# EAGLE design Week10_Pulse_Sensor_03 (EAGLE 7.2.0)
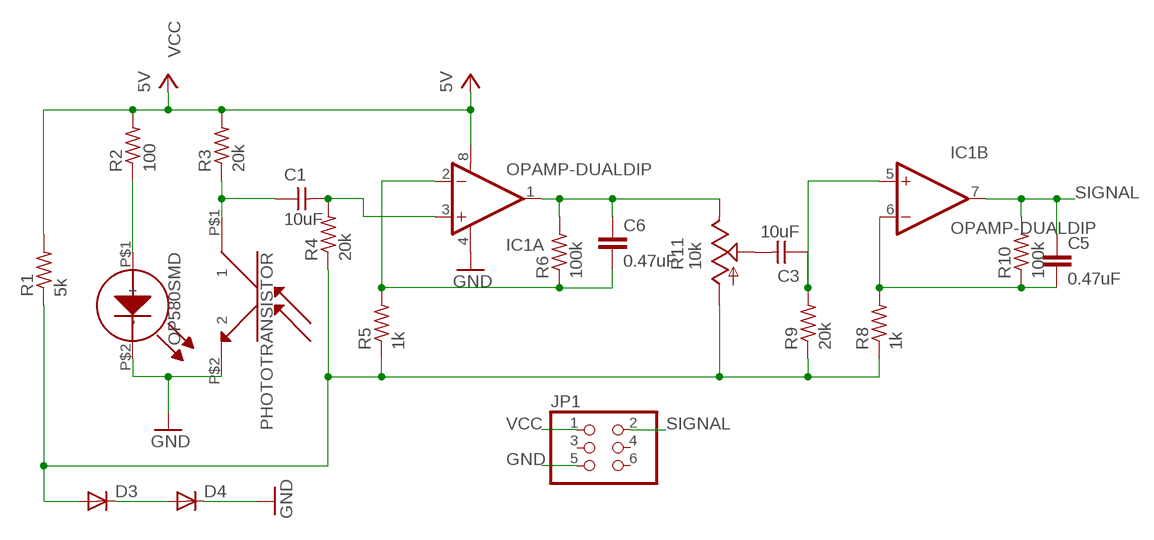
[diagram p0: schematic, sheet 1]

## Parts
C1  10uF  UNPOLARIZED_CAPACITOR1206  [1206]
C3  10uF  UNPOLARIZED_CAPACITOR1206  [1206]
C5  0.47uF  C-EU050-045X075  [C050-045X075]
C6  0.47uF  C-EU050-045X075  [C050-045X075]
D3  DIODESOD123  [SOD123]
D4  DIODESOD123  [SOD123]
IC1  OPAMP-DUALDIP  [DIP08]
JP1  PINHD-2X3-SMD  [2X03SMD]
LED  OP280SMD  [OP280]
PHOTOTRANSISTOR  OP580SMD  [OP580]
R1  5k  RES-US1206FAB  [R1206FAB]
R2  100  RES-US1206FAB  [R1206FAB]
R3  20k  RES-US1206FAB  [R1206FAB]
R4  20k  RES-US1206FAB  [R1206FAB]
R5  1k  RES-US1206FAB  [R1206FAB]
R6  100k  RES-US1206FAB  [R1206FAB]
R8  1k  RES-US1206FAB  [R1206FAB]
R9  20k  RES-US1206FAB  [R1206FAB]
R10  100k  RES-US1206FAB  [R1206FAB]
R11  10k  TRIM_US-S64W  [S64W]

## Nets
GND: D4.CATHODE(C) IC1.4(A:V-) JP1.5 LED.P$2(-) PHOTOTRANSISTOR.P$2
N$1: C1.1 PHOTOTRANSISTOR.P$1 R3.1
N$2: LED.P$1(+) R2.1
N$3: D3.CATHODE(C) D4.ANODE(A)
N$4: C5.2 IC1.6(B:-IN) R8.2 R10.1
N$5: C6.2 IC1.2(A:-IN) R5.2 R6.1
N$6: C1.2 IC1.3(A:+IN) R4.2
N$7: C6.1 IC1.1(A:OUT) R6.2 R11.E
N$8: C3.2 R11.S
N$9: C3.1 IC1.5(B:+IN) R9.2
N$11: D3.ANODE(A) R1.1 R4.1 R5.1 R8.1 R9.1 R11.A
SIGNAL: C5.1 IC1.7(B:OUT) JP1.2 R10.2
VCC: IC1.8(A:V+) JP1.1 R1.2 R2.2 R3.2 ; supply symbol labelled 5V
Unconnected: JP1.3 JP1.4 JP1.6

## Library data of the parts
C1 C3 = 01_ng:UNPOLARIZED_CAPACITOR: unpolarized_capacitor
C5 C6 = rcl:C-EU: CAPACITOR, European symbol
D3 D4 = 01_fab:DIODE: DIODE
IC1 = SparkFun-AnalogIC:OPAMP-DUAL: Generic op-amp footprint
JP1 = 01_FAB_Hello:PINHD-2X3-SMD: PIN HEADER
LED = Optics:OP280
PHOTOTRANSISTOR = Optics:OP580
R1-R6 R8-R10 = 01_fab:RES-US: Resistor (US Symbol)
R11 = pot:TRIM_US-: POTENTIOMETER

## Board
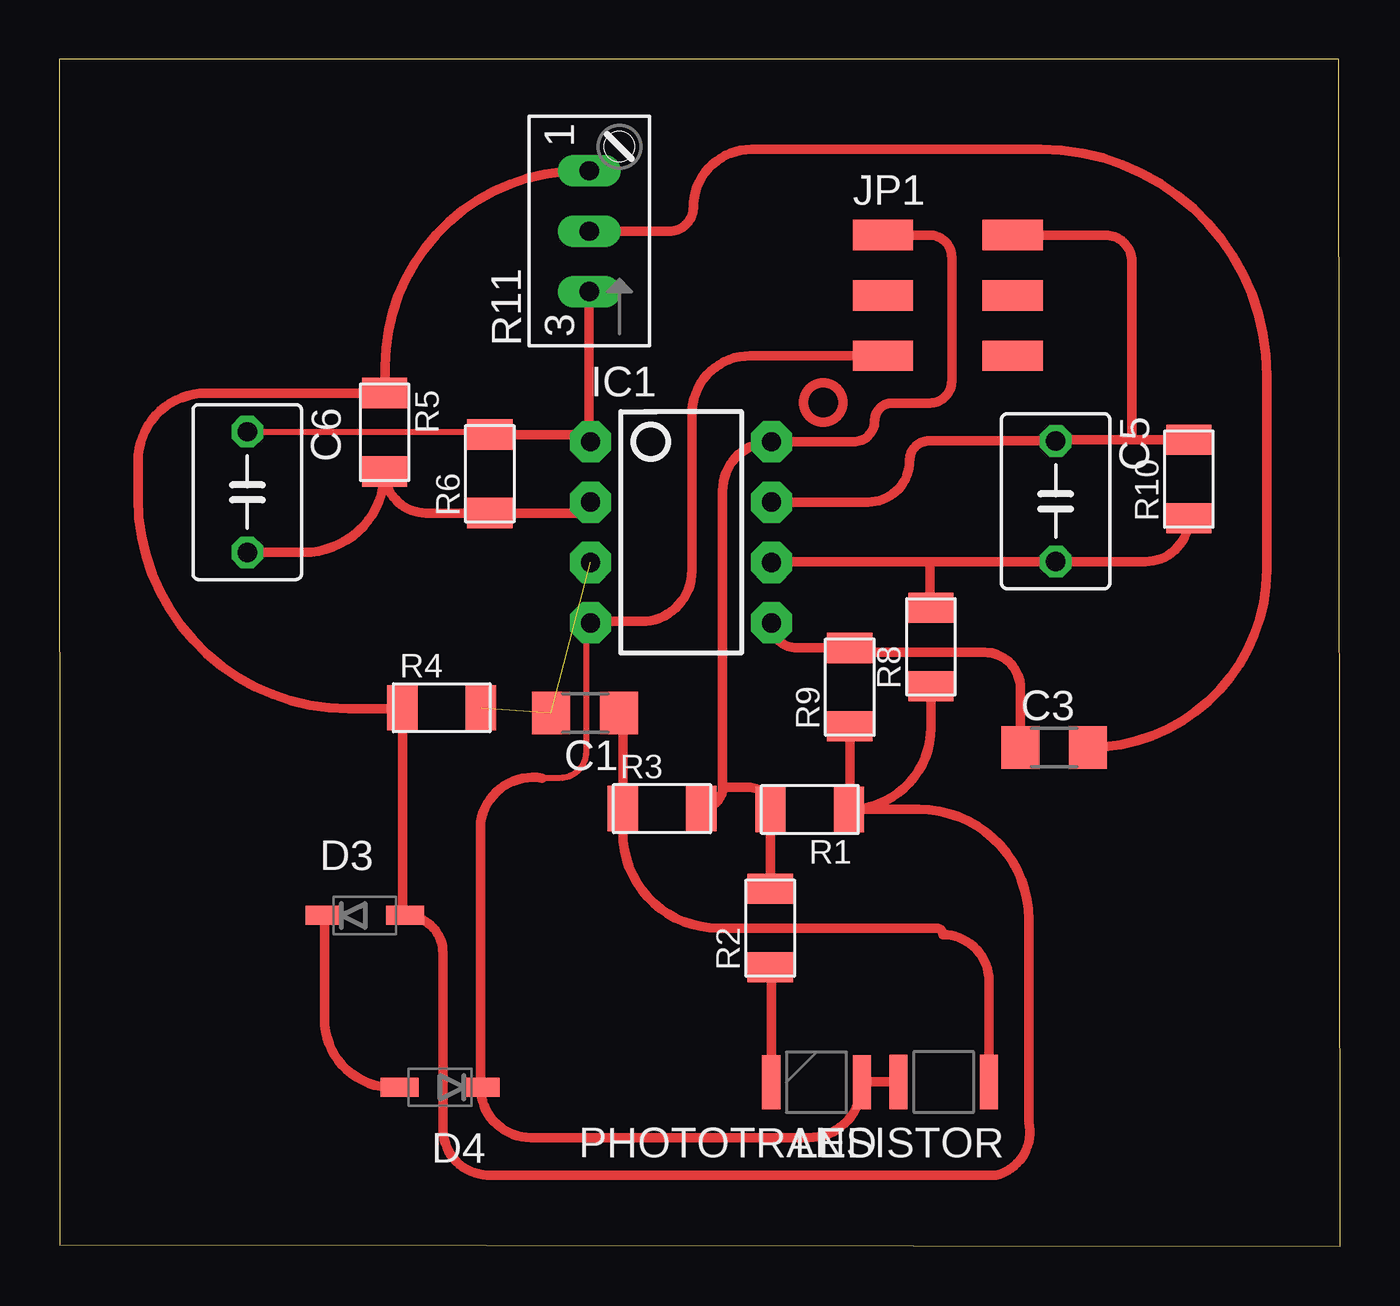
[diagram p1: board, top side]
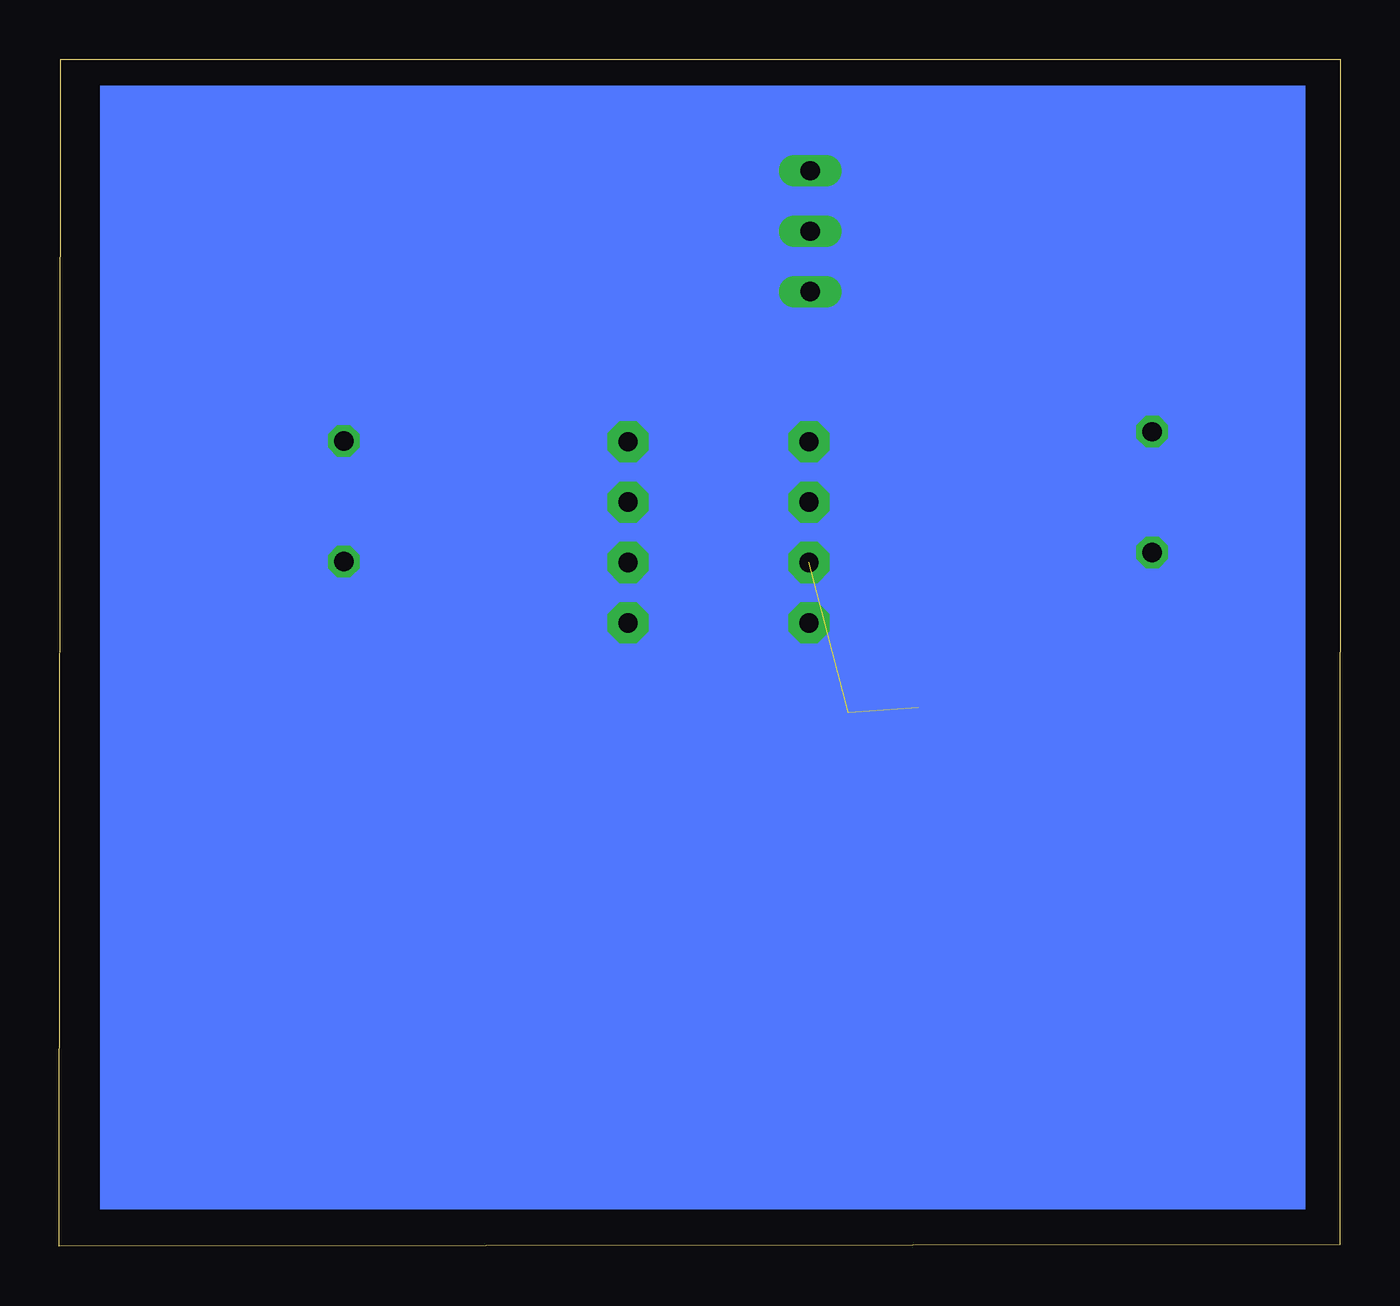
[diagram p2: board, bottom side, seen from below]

Size 53.91 x 49.95 mm. Coordinates in mm from the lower left corner, seen from the top.
Outline: 0.01,0.08 53.91,0 53.85,49.95 0,49.95 0.01,0.08
Copper layers (1*16): Top 0.035mm / dielectric 1.5mm / Bottom 0.035mm
Design rules "fabmodule": minimum track width 10mil, minimum drill 0.4mm, track to track 0.42mm, track to pad 0.42mm, pad to pad 0.42mm, via to via 0.42mm, smd to smd 0.42mm, copper to edge 40mil, drill to drill 0.8mm, minimum pad ring 10mil, minimum via ring 8mil, stop-mask expansion 4mil, vias tented up to drill 0mil, thermal gap 10mil

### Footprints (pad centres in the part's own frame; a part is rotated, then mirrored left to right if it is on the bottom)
1206 = smd 1.6 x 1.803: 1 -1.422,0; 2 1.422,0
C050-045X075 = drill 0.813 octagon: 1 -2.54,0; 2 2.54,0
SOD123 = smd 1.6 x 0.8: ANODE 1.7,0; CATHODE -1.7,0
DIP08 = drill 0.813 pad 1.727 octagon: 1 -3.81,-3.81; 2 -1.27,-3.81; 3 1.27,-3.81; 4 3.81,-3.81; 5 3.81,3.81; 6 1.27,3.81; 7 -1.27,3.81; 8 -3.81,3.81
2X03SMD = smd 2.54 x 1.27: 1 -2.54,2.54; 2 2.92,2.54; 3 -2.54,0; 4 2.92,0; 5 -2.54,-2.54; 6 2.92,-2.54
OP280 = smd 0.762 x 2.286: P$1 1.905,0; P$2 -1.905,0
OP580 = smd 0.762 x 2.286: P$1 -1.905,0; P$2 1.905,0
R1206FAB = smd 1.27 x 1.905: 1 -1.651,0; 2 1.651,0
S64W = drill 0.813 long: A 2.54,1.27; E -2.54,1.27; S 0,1.27

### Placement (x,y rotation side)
C1  22.13,22.45 180 top
C3  41.87,21 0 top
C5  41.94,31.36 270 top
C6  7.91,31.74 270 top
D3  12.86,13.93 0 top
D4  16.03,6.7 180 top
IC1  26.17,30.05 270 top
JP1  37.2,40.02 0 top
LED  31.87,6.91 180 top
PHOTOTRANSISTOR  37.22,6.92 180 top
R1  31.59,18.39 180 top
R2  29.92,13.4 90 top
R3  25.37,18.42 0 top
R4  16.09,22.67 0 top
R5  13.69,34.26 270 top
R6  18.12,32.51 90 top
R8  36.68,25.23 90 top
R9  33.27,23.53 90 top
R10  47.54,32.29 90 top
R11  23.57,42.72 90 top

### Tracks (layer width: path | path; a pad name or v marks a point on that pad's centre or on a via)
GND
  Top 0.254: 22.08,26.76 arc-90 22.17,26.67 22.17,20.82 arc-90 21.06,19.71 20.32,19.71
  Top 0.406: JP1.5 29.08,37.48 arc90 26.62,35.02 26.62,28.43 arc-90 24.49,26.3 22.41,26.3 arc90 IC1.4 22.36,26.49 arc90 22.08,26.76 | 20.32,19.71 arc90 17.73,17.86 D4.CATHODE arc90 19.85,4.58 31.54,4.58 arc90 33.77,6.82 LED.P$2 arc-90 33.79,6.92 PHOTOTRANSISTOR.P$2
N$1
  Top 0.406: C1.1 arc-90 23.72,22.28 R3.1 23.72,17.42 arc90 27.74,13.4 36.91,13.4 arc-90 37.19,13.12 arc-90 39.13,11.18 PHOTOTRANSISTOR.P$1
N$2
  Top 0.406: R2.1 arc-90 29.96,11.7 LED.P$1
N$3
  Top 0.406: D3.CATHODE 11.16,9.31 arc90 D4.ANODE
N$4
  Top 0.406: IC1.6 29.98,28.82 36.64,28.82 | 36.64,28.82 C5.2 45.72,28.82 arc90 R10.1 | R8.2 arc-90 36.64,26.93 36.64,28.82
N$5
  Top 0.406: IC1.2 arc-90 21.9,30.86 R6.1 15.44,30.86 arc-90 R5.2 arc-90 10.28,29.2 C6.2
N$6  (2 unrouted)
N$7
  Top 0.254: C6.1 18,34.28 arc-90 R6.2
  Top 0.406: 22.05,34.16 arc-90 IC1.1 | 22.32,33.9 arc90 IC1.1 | R11.E 22.3,33.91 arc90 IC1.1 | 17.87,34.16 arc-90 R6.2 22.05,34.16 | 22.05,34.16 arc-90 IC1.1
N$8
  Top 0.406: R11.S 25.68,42.72 arc90 26.68,43.72 arc-90 29.13,46.17 41.31,46.17 arc-90 50.83,36.65 50.83,28.47 arc-90 C3.2
N$9
  Top 0.406: IC1.5 arc90 31.03,25.19 R9.2 arc90 33.46,25 38.95,25 arc-90 40.45,23.5 C3.1
N$11
  Top 0.406: R11.A 21.94,45.26 arc90 13.71,37.03 13.71,35.94 arc-90 R5.1 6.18,35.91 arc90 3.31,33.05 3.31,31.49 arc90 12.17,22.63 14.4,22.63 arc90 R4.1 14.44,14.05 arc90 D3.ANODE arc-90 16.15,12.34 16.15,4.86 arc90 18.19,3 39.42,3 arc90 40.81,5.23 40.81,13.77 arc90 36.18,18.39 R1.1 | R1.1 arc90 33.27,18.42 R9.1 | R1.1 arc90 36.68,21.84 R8.1
SIGNAL
  Top 0.406: 45.15,33.94 41.72,33.94 arc90 C5.1 36.61,33.9 arc90 35.79,33.07 arc-90 34.04,31.32 IC1.7 | 45.15,33.94 R10.2 | 45.15,33.94 45.15,41.43 arc90 44.02,42.56 JP1.2
VCC
  Top 0.406: JP1.1 36.62,42.56 arc-90 37.56,41.61 37.56,36.42 arc-90 36.64,35.49 35.06,35.49 arc90 34.32,34.75 arc-90 33.43,33.86 IC1.8 arc90 27.92,31.81 27.92,19.33 | 27.92,19.33 arc-90 R3.2 | 27.92,19.33 29,19.33 arc-90 R1.2 29.94,15.07 arc-90 R2.2
(copper drawn outside any net)
  shapes: Bottom area x1, Top circle x1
